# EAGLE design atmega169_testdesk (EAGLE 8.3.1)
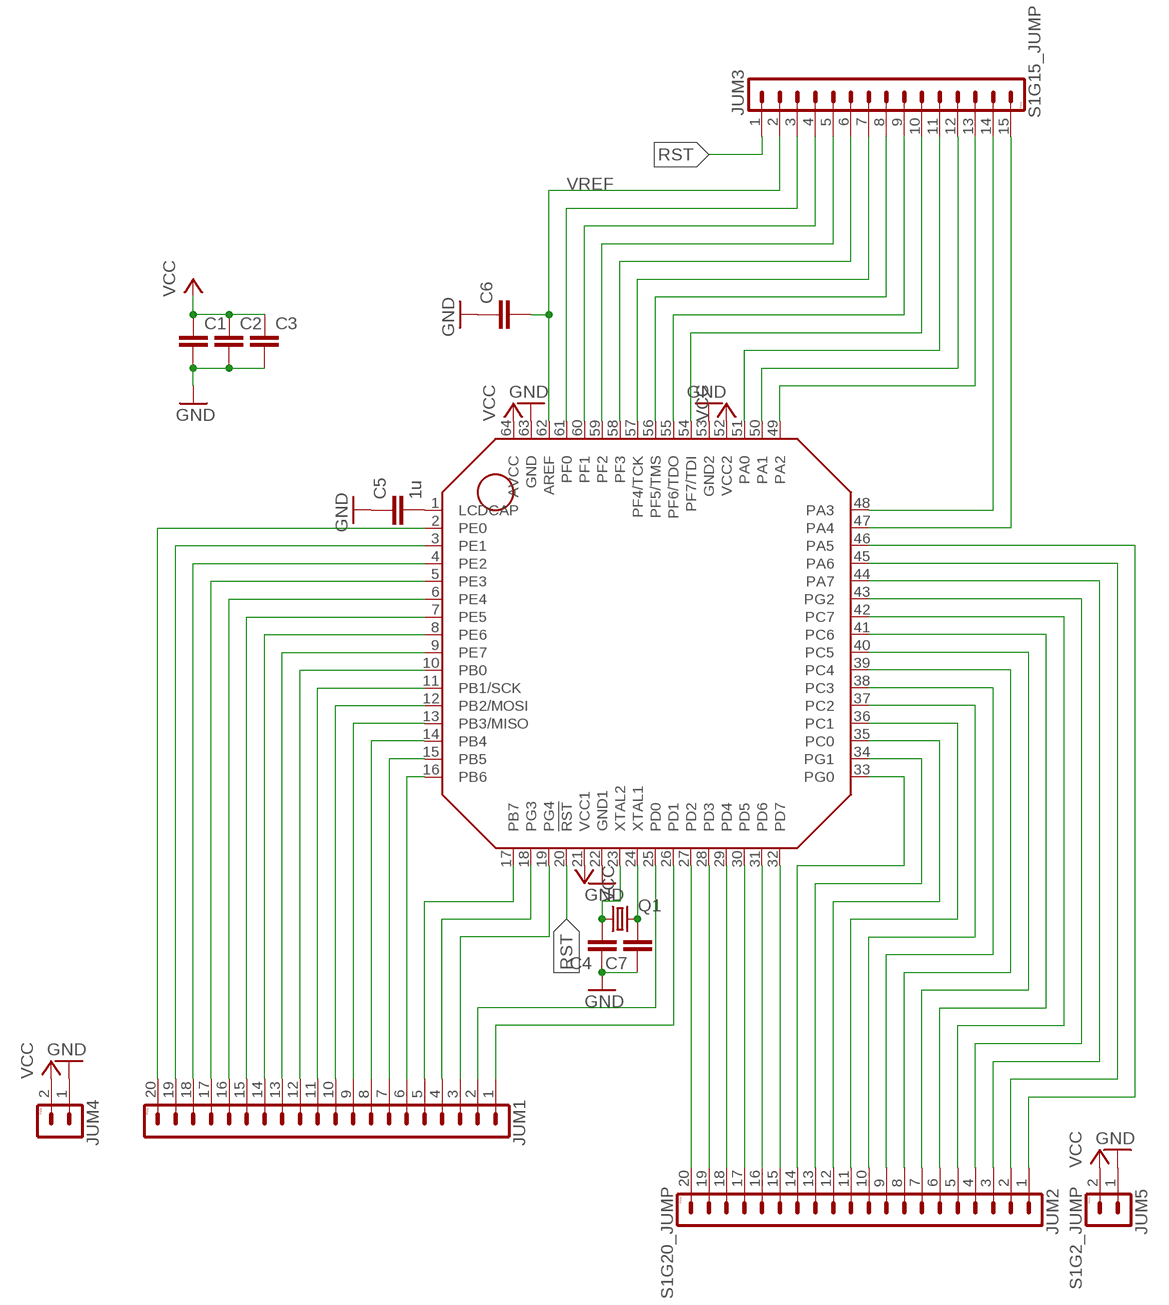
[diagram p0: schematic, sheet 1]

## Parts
C1  C-EUC0603  [C0603]
C2  C-EUC0603  [C0603]
C3  C-EUC0603  [C0603]
C4  C-EUC0603  [C0603]
C5  1u  C-EUC0603  [C0603]
C6  C-EUC0603  [C0603]
C7  C-EUC0603  [C0603]
JUM1  S1G20_JUMP  [S1G20_JU]
JUM2  S1G20_JUMP  [S1G20_JU]
JUM3  S1G15_JUMP  [S1G15_JU]
JUM4  S1G2_JUMP  [S1G2_JUM]
JUM5  S1G2_JUMP  [S1G2_JUM]
Q1  CRYSTALTC26V  [TC26V]
U$1  ATMEGA169-16A  [TQFP64]

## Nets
GND: C1.2 C2.2 C3.2 C4.1 C5.1 C6.1 C7.1 JUM4.1 JUM5.1 U$1.22(GND1) U$1.53(GND2) U$1.63(GND)
N$2: C5.2 U$1.1(LCDCAP)
N$20: C4.2 Q1.1 U$1.23(XTAL2)
N$21: C7.2 Q1.2 U$1.24(XTAL1)
PA0: JUM3.11 U$1.51(PA0)
PA1: JUM3.12 U$1.50(PA1)
PA2: JUM3.13 U$1.49(PA2)
PA3: JUM3.14 U$1.48(PA3)
PA4: JUM3.15 U$1.47(PA4)
PA5: JUM2.1 U$1.46(PA5)
PA6: JUM2.2 U$1.45(PA6)
PA7: JUM2.3 U$1.44(PA7)
PB0: JUM1.12 U$1.10(PB0)
PB1/SCK: JUM1.11 U$1.11(PB1/SCK)
PB2/MOSI: JUM1.10 U$1.12(PB2/MOSI)
PB3/MISO: JUM1.9 U$1.13(PB3/MISO)
PB4: JUM1.8 U$1.14(PB4)
PB5: JUM1.7 U$1.15(PB5)
PB6: JUM1.6 U$1.16(PB6)
PB7: JUM1.5 U$1.17(PB7)
PC0: JUM2.12 U$1.35(PC0)
PC1: JUM2.11 U$1.36(PC1)
PC2: JUM2.10 U$1.37(PC2)
PC3: JUM2.9 U$1.38(PC3)
PC4: JUM2.8 U$1.39(PC4)
PC5: JUM2.7 U$1.40(PC5)
PC6: JUM2.6 U$1.41(PC6)
PC7: JUM2.5 U$1.42(PC7)
PD0: JUM1.2 U$1.25(PD0)
PD1: JUM1.1 U$1.26(PD1)
PD2: JUM2.20 U$1.27(PD2)
PD3: JUM2.19 U$1.28(PD3)
PD4: JUM2.18 U$1.29(PD4)
PD5: JUM2.17 U$1.30(PD5)
PD6: JUM2.16 U$1.31(PD6)
PD7: JUM2.15 U$1.32(PD7)
PE0: JUM1.20 U$1.2(PE0)
PE1: JUM1.19 U$1.3(PE1)
PE2: JUM1.18 U$1.4(PE2)
PE3: JUM1.17 U$1.5(PE3)
PE4: JUM1.16 U$1.6(PE4)
PE5: JUM1.15 U$1.7(PE5)
PE6: JUM1.14 U$1.8(PE6)
PE7: JUM1.13 U$1.9(PE7)
PF0: JUM3.3 U$1.61(PF0)
PF1: JUM3.4 U$1.60(PF1)
PF2: JUM3.5 U$1.59(PF2)
PF3: JUM3.6 U$1.58(PF3)
PF4/TCK: JUM3.7 U$1.57(PF4/TCK)
PF5/TMS: JUM3.8 U$1.56(PF5/TMS)
PF6/TDO: JUM3.9 U$1.55(PF6/TDO)
PF7/TDI: JUM3.10 U$1.54(PF7/TDI)
PG0: JUM2.14 U$1.33(PG0)
PG1: JUM2.13 U$1.34(PG1)
PG2: JUM2.4 U$1.43(PG2)
PG3: JUM1.4 U$1.18(PG3)
PG4: JUM1.3 U$1.19(PG4)
RST: JUM3.1 U$1.20(!RST!)
VCC: C1.1 C2.1 C3.1 JUM4.2 JUM5.2 U$1.21(VCC1) U$1.52(VCC2) U$1.64(AVCC)
VREF: C6.2 JUM3.2 U$1.62(AREF)

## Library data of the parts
C1-C7 = rcl:C-EU: CAPACITOR, European symbol
JUM1 JUM2 = PaJa_konektory:S1G20_JUMP: Radove konektory - koliky - 20x
JUM3 = PaJa_konektory:S1G15_JUMP: Radove konektory - koliky - 15x
JUM4 JUM5 = PaJa_konektory:S1G2_JUMP: Radove konektory - koliky - 2x
Q1 = crystal:CRYSTAL: CRYSTAL; OC_FARNELL: unknown; OC_NEWARK: unknown
U$1 = atmel:ATMEGA169: 8-bit Microcontroller with 16K Flash, LCD driver, JTAG

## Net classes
0 default: width 0.305 mm, drill 0.9 mm, clearance 0.254 mm

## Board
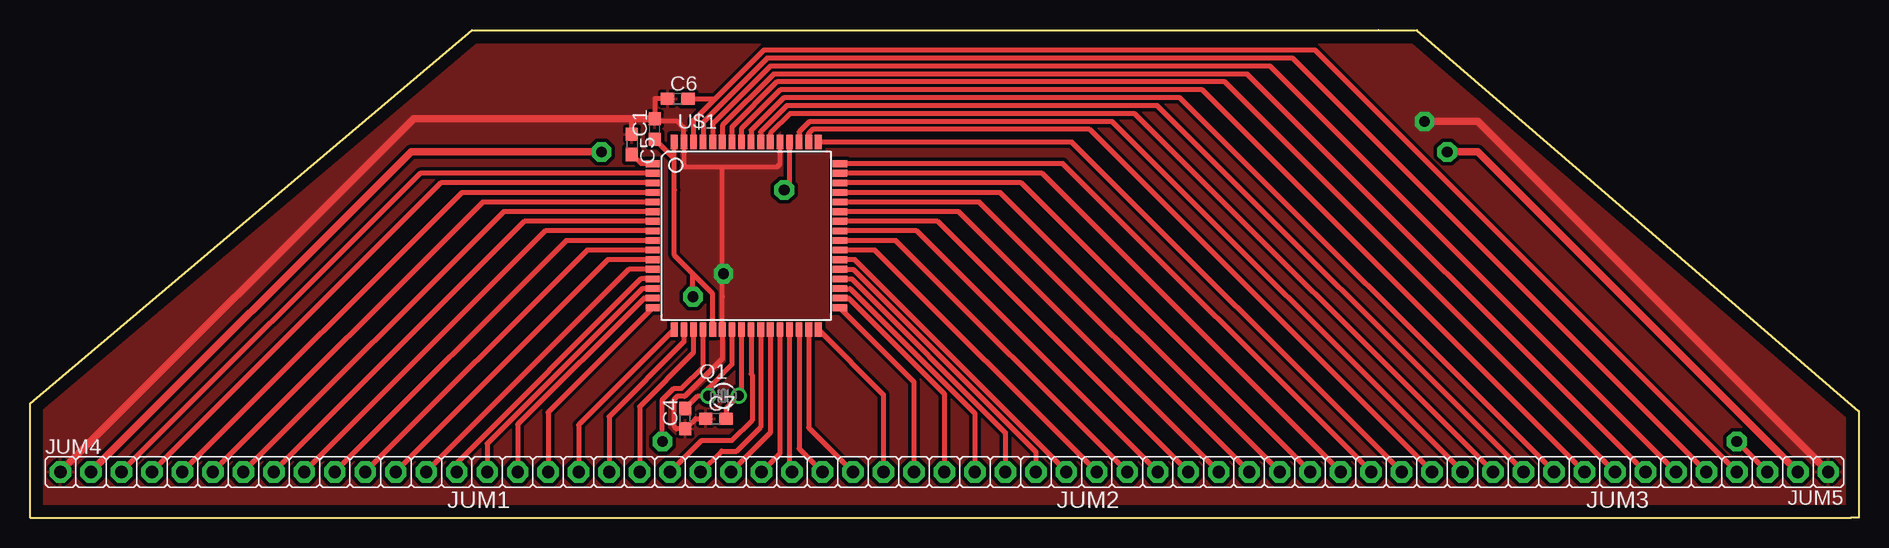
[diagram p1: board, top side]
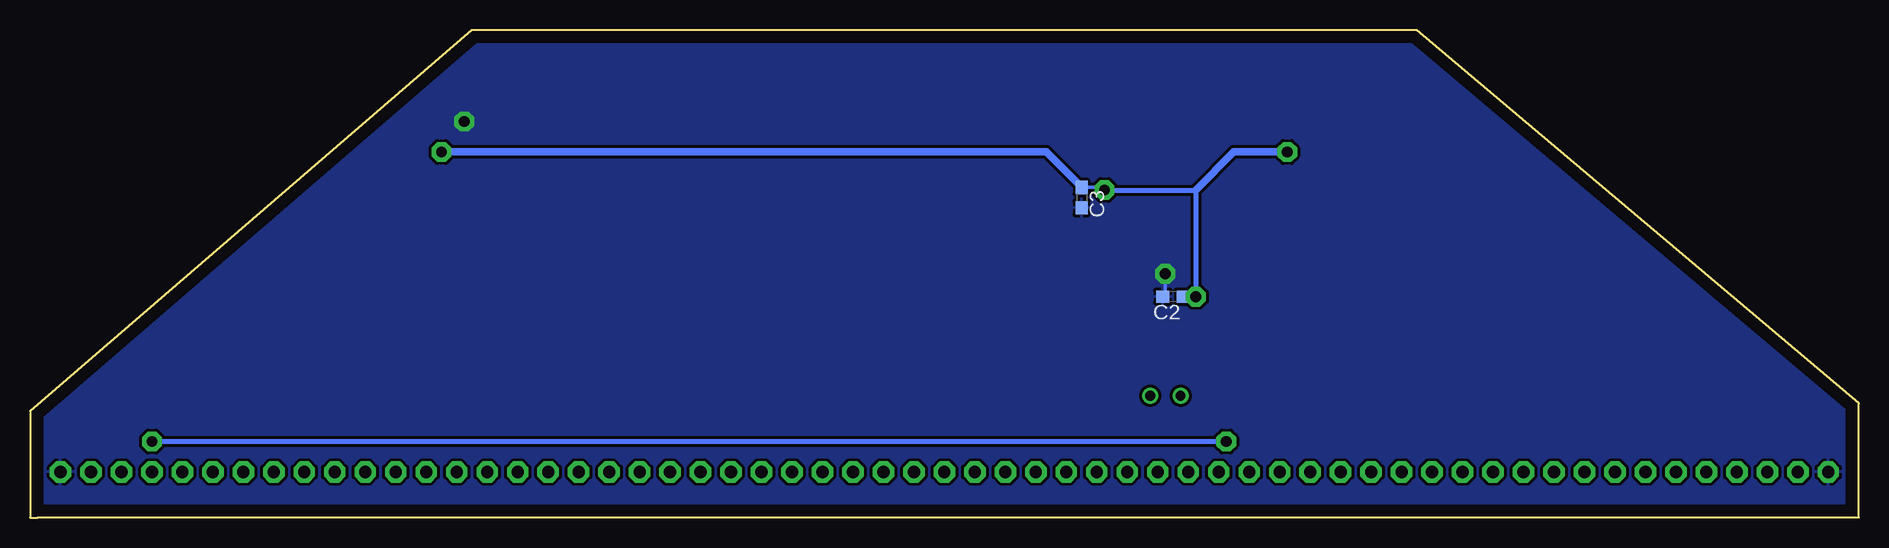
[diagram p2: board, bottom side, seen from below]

Size 152.4 x 40.64 mm. Coordinates in mm from the lower left corner, seen from the top.
Outline: 151.76,0 151.79,0
Outline: 151.76,0 152.4,0 152.4,8.89 115.57,40.64 112.39,40.64 36.83,40.64 0,9.53 0,0 151.76,0
Copper layers (1*16): Top 0.035mm / dielectric 1.5mm / Bottom 0.035mm
Design rules "default": minimum track width 6mil, minimum drill 0.35mm, track to track 6mil, track to pad 6mil, pad to pad 6mil, via to via 6mil, smd to smd 6mil, copper to edge 40mil, drill to drill 6mil, minimum pad ring 10mil, minimum via ring 8mil, stop-mask expansion 4mil, vias tented up to drill 0mil, thermal gap 10mil

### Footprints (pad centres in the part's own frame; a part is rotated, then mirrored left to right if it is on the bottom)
C0603 = smd 1.1 x 1: 1 -0.85,0; 2 0.85,0
S1G20_JU = drill 1.016 pad 1.778 octagon: 1 -24.13,0; 2 -21.59,0; 3 -19.05,0; 4 -16.51,0; 5 -13.97,0; 6 -11.43,0; 7 -8.89,0; 8 -6.35,0; 9 -3.81,0; 10 -1.27,0; 11 1.27,0; 12 3.81,0; 13 6.35,0; 14 8.89,0; 15 11.43,0; 16 13.97,0; 17 16.51,0; 18 19.05,0; 19 21.59,0; 20 24.13,0
S1G15_JU = drill 1.016 pad 1.778 octagon: 1 -17.78,0; 2 -15.24,0; 3 -12.7,0; 4 -10.16,0; 5 -7.62,0; 6 -5.08,0; 7 -2.54,0; 8 0,0; 9 2.54,0; 10 5.08,0; 11 7.62,0; 12 10.16,0; 13 12.7,0; 14 15.24,0; 15 17.78,0
S1G2_JUM = drill 1.016 pad 1.778 octagon: 1 -1.27,0; 2 1.27,0
TC26V = drill 0.813: 1 -1.27,0; 2 1.27,0
TQFP64 = smd 1.194 x 0.559: 1 -7.8,6; 2 -7.8,5.2; 3 -7.8,4.4; 4 -7.8,3.6; 5 -7.8,2.8; 6 -7.8,2; 7 -7.8,1.2; 8 -7.8,0.4; 9 -7.8,-0.4; 10 -7.8,-1.2; 11 -7.8,-2; 12 -7.8,-2.8; 13 -7.8,-3.6; 14 -7.8,-4.4; 15 -7.8,-5.2; 16 -7.8,-6; 33 7.8,-6; 34 7.8,-5.2; 35 7.8,-4.4; 36 7.8,-3.6; 37 7.8,-2.8; 38 7.8,-2; 39 7.8,-1.2; 40 7.8,-0.4; 41 7.8,0.4; 42 7.8,1.2; 43 7.8,2; 44 7.8,2.8; 45 7.8,3.6; 46 7.8,4.4; 47 7.8,5.2; 48 7.8,6 | smd 0.559 x 1.194: 17 -6,-7.8; 18 -5.2,-7.8; 19 -4.4,-7.8; 20 -3.6,-7.8; 21 -2.8,-7.8; 22 -2,-7.8; 23 -1.2,-7.8; 24 -0.4,-7.8; 25 0.4,-7.8; 26 1.2,-7.8; 27 2,-7.8; 28 2.8,-7.8; 29 3.6,-7.8; 30 4.4,-7.8; 31 5.2,-7.8; 32 6,-7.8; 49 6,7.8; 50 5.2,7.8; 51 4.4,7.8; 52 3.6,7.8; 53 2.8,7.8; 54 2,7.8; 55 1.2,7.8; 56 0.4,7.8; 57 -0.4,7.8; 58 -1.2,7.8; 59 -2,7.8; 60 -2.8,7.8; 61 -3.6,7.8; 62 -4.4,7.8; 63 -5.2,7.8; 64 -6,7.8

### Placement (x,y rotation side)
C1  52.07,32.38 90 top
C2  57.15,18.41 180 bottom
C3  64.77,26.67 270 bottom
C4  54.61,8.26 90 top
C5  50.16,31.11 270 top
C6  53.98,34.92 0 top
C7  57.15,8.26 0 top
JUM1  31.75,3.81 180 top
JUM2  82.55,3.81 180 top
JUM3  127,3.81 180 top
JUM4  3.81,3.81 0 top
JUM5  148.59,3.81 180 top
Q1  57.78,10.16 0 top
U$1  59.69,23.5 0 top

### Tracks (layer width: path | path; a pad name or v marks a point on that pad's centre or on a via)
GND  (via drill 0.9 pad 1.65)
  Top 0.305: v57.78,20.32 57.69,20.32
  Top 0.406: U$1.53 62.49,29.47 62.23,29.21 60.33,29.21 57.78,29.21 | 57.78,29.21 54.61,29.21 54.49,29.33 U$1.63 54.49,32.51 53.98,33.02 52.28,33.02 C1.2 | 57.78,29.21 57.69,29.11 57.69,20.32 57.69,18.41 U$1.22 57.69,13.24 54.56,10.11 53.92,10.11 53.65,9.84 53.65,7.62 53.87,7.41 C4.1 55.46,8.26 C7.1 | C5.1 50.16,33.02 50.38,33.23 C1.2 | C6.1 52.07,34.92 C1.2
  Top 0.61: JUM4.1 31.96,33.23 C1.2 | JUM5.1 120.65,33.02 v116.2,33.02
  Bottom 0.305: v57.78,20.32 57.78,18.63 C2.2
  pour Top (isolate 0.305): 0,9.53 0,0 152.4,0 152.4,8.89 120.65,40.64 31.11,40.64
  pour Bottom (isolate 0.254): 0,0 152.4,0 152.4,9.53 121.28,40.64 31.75,40.64 0,8.89
N$2
  Top 0.406: U$1.1 50.94,29.5 C5.2
N$20
  Top 0.406: U$1.23 58.49,12.77 56.52,10.79 Q1.1 55.66,10.16 C4.2
N$21
  Top 0.406: U$1.24 59.29,10.39 Q1.2 58,9.11 C7.2
PA0
  Top 0.406: JUM3.11 90.18,33.01 64.95,33.01 64.09,32.15 U$1.51
PA1
  Top 0.406: JUM3.12 88.3,32.35 65.22,32.35 64.89,32.02 U$1.50
PA2
  Top 0.406: JUM3.13 86.81,31.3 U$1.49
PA3
  Top 0.406: JUM3.14 86.08,29.5 U$1.48
PA4
  Top 0.406: JUM3.15 84.33,28.7 U$1.47
PA5
  Top 0.406: JUM2.1 82.59,27.89 U$1.46
PA6
  Top 0.406: JUM2.2 80.86,27.09 U$1.45
PA7
  Top 0.406: JUM2.3 79.11,26.3 U$1.44
PB0
  Top 0.406: U$1.10 46.42,22.3 JUM1.12
PB1/SCK
  Top 0.406: U$1.11 48.16,21.5 JUM1.11
PB2/MOSI
  Top 0.406: U$1.12 49.91,20.7 JUM1.10
PB3/MISO
  Top 0.406: U$1.13 50.9,19.89 35.56,4.56 JUM1.9
PB4
  Top 0.406: U$1.14 51.03,19.09 38.1,6.16 JUM1.8
PB5
  Top 0.406: U$1.15 51.17,18.3 40.64,7.77 JUM1.7
PB6
  Top 0.406: U$1.16 43.18,8.79 JUM1.6
PB7
  Top 0.406: U$1.17 45.72,7.72 JUM1.5
PC0
  Top 0.406: U$1.35 68.35,19.09 78.74,8.7 JUM2.12
PC1
  Top 0.406: U$1.36 68.48,19.89 81.28,7.1 JUM2.11
PC2
  Top 0.406: U$1.37 68.61,20.7 83.82,5.49 JUM2.10
PC3
  Top 0.406: JUM2.9 86.36,3.88 68.75,21.5 U$1.38
PC4
  Top 0.406: JUM2.8 70.42,22.3 U$1.39
PC5
  Top 0.406: JUM2.7 72.16,23.09 U$1.40
PC6
  Top 0.406: JUM2.6 73.89,23.89 U$1.41
PC7
  Top 0.406: JUM2.5 75.64,24.7 U$1.42
PD0
  Top 0.406: U$1.25 60.09,11.98 60.17,11.89 60.17,8.1 58.49,6.41 55.94,6.41 JUM1.2
PD1
  Top 0.406: U$1.26 60.89,7.55 58.9,5.55 57.62,5.55 JUM1.1
PD2
  Top 0.406: U$1.27 61.69,7.08 JUM2.20
PD3
  Top 0.406: U$1.28 62.49,5.34 JUM2.19
PD4
  Top 0.406: U$1.29 63.29,4.02 JUM2.18
PD5
  Top 0.406: U$1.30 64.09,5.76 JUM2.17
PD6
  Top 0.406: U$1.31 64.89,7.5 JUM2.16
PD7
  Top 0.406: U$1.32 71.12,10.27 JUM2.15
PE0
  Top 0.406: U$1.2 32.51,28.7 JUM1.20
PE1
  Top 0.406: U$1.3 34.24,27.89 JUM1.19
PE2
  Top 0.406: U$1.4 35.98,27.09 JUM1.18
PE3
  Top 0.406: U$1.5 37.73,26.3 JUM1.17
PE4
  Top 0.406: U$1.6 39.47,25.5 JUM1.16
PE5
  Top 0.406: U$1.7 41.2,24.7 JUM1.15
PE6
  Top 0.406: U$1.8 42.95,23.89 JUM1.14
PE7
  Top 0.406: U$1.9 44.69,23.09 JUM1.13
PF0
  Top 0.406: JUM3.3 105.22,38.29 61.43,38.29 56.09,32.96 U$1.61
PF1
  Top 0.406: JUM3.4 103.34,37.63 61.7,37.63 56.89,32.82 U$1.60
PF2
  Top 0.406: JUM3.5 101.46,36.97 61.97,36.97 57.69,32.69 U$1.59
PF3
  Top 0.406: JUM3.6 99.58,36.31 62.25,36.31 58.49,32.55 U$1.58
PF4/TCK
  Top 0.406: JUM3.7 97.7,35.65 62.52,35.65 59.29,32.42 U$1.57
PF5/TMS
  Top 0.406: JUM3.8 95.82,34.99 62.8,34.99 60.09,32.29 U$1.56
PF6/TDO
  Top 0.406: JUM3.9 93.94,34.33 63.07,34.33 60.89,32.15 U$1.55
PF7/TDI
  Top 0.406: JUM3.10 92.06,33.67 63.34,33.67 61.69,32.02 U$1.54
PG0
  Top 0.406: U$1.33 73.66,11.32 JUM2.14
PG1
  Top 0.406: U$1.34 68.21,18.3 76.2,10.31 JUM2.13
PG2
  Top 0.406: JUM2.4 77.38,25.5 U$1.43
PG3
  Top 0.406: U$1.18 54.49,14.66 48.26,8.43 JUM1.4
PG4
  Top 0.406: U$1.19 55.29,13.75 50.8,9.26 JUM1.3
RST  (via drill 0.9 pad 1.65)
  Top 0.406: JUM3.1 v142.24,6.35 | v52.7,6.35 52.7,9.83 53.65,10.77 54.29,10.77 56.09,12.57 U$1.20
  Bottom 0.406: v142.24,6.35 v52.7,6.35
VCC  (via drill 0.9 pad 1.65)
  Top 0.406: 53.69,29.91 53.69,27.3 53.69,21.88 55.24,20.32 | 53.69,29.91 U$1.64 | U$1.21 56.89,18.68 55.24,20.32 | U$1.52 63.29,27.73 v62.87,27.3 | C1.1 53.69,29.91 | v55.24,18.41 55.24,20.32
  Top 0.61: JUM4.2 31.75,30.48 v47.62,30.48 | JUM5.2 120.65,30.48 v118.11,30.48
  Bottom 0.305: C3.1 63.08,27.52 v62.87,27.3
  Bottom 0.406: v62.87,27.3 55.24,27.3 v55.24,18.41 C2.1
  Bottom 0.61: v47.62,30.48 52.07,30.48 55.24,27.3 | v118.11,30.48 67.73,30.48 C3.1
VREF
  Top 0.406: JUM3.2 107.1,38.95 61.15,38.95 57.14,34.94 | 57.14,34.94 55.29,33.09 U$1.62 | C6.2 57.12,34.92 57.14,34.94

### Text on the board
tDocu: GND | VCC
